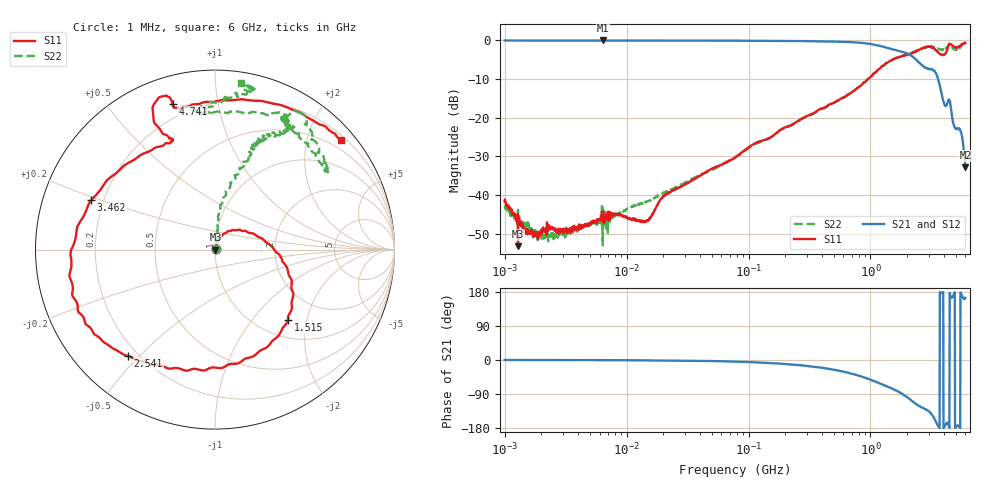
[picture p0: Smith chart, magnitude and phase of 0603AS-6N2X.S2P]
!s-Parameter Generated by FASTRON Sdn. Bhd.
!FASTRON P/N : 0603AS-6N2X
!Keysight Technologies: E5071C_MY46733604_B.14.02
!Date: Tue Nov 21 15:09:04 2023
!Version  :Rev01  Tue Nov 21 15:09:04 2023
!Data & Calibration Information:
!Freq  S11:SOLT2(ON)  S21:SOLT2(ON)  S12:SOLT2(ON)  S22:SOLT2(ON)
!PortZ  Port1:50+j0  Port2:50+j0
!When reading reference impedance value at option line is always used.
! Remarks : This data is being provided solely for informational purposes.
# Hz S dB R 50
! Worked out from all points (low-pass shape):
!   1601 points, 1 MHz to 6 GHz, reference 50 ohm
!   highest |S21| = -0.01 dB at 6.378 MHz (marker M1); lowest = -32.8 dB at 6 GHz (marker M2)
!   |S21| within 3 dB of the highest: start of sweep to 1.829 GHz
!   lowest |S11| = -53.2 dB at 1.288 MHz (marker M3), VSWR 1.00, Z = 50.2 - j0.0158 ohm
!   |S11| at or under -10 dB: start of sweep to 953.5 MHz
!   |S22| runs from -53.0 to -0.5 dB; largest |S21 - S12| = 0.01
!   S11 on the Smith chart (normalised r, x): 1 MHz: 1.02, +0.01; 1.515 GHz: 1.35, -1.55; 2.541 GHz: 0.16, -0.46; 3.462 GHz: 0.15, +0.19; 4.741 GHz: 0.13, +0.74; 6 GHz: 0.30, +2.64
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1000000  -41.61 20.7  -0.03 0.1  -0.05 0.2  -42.82 27.1
1287650  -53.18 -4.1  -0.05 -0.0  -0.04 0.1  -43.78 5.1
2105185  -49.18 39.2  -0.04 -0.1  -0.05 -0.0  -50.93 47.0
4277066  -48.43 44.9  -0.04 -0.2  -0.04 -0.2  -48.53 52.3
6378092  -46.48 62.7  -0.01 -0.4  -0.07 -0.5  -52.95 65.8
1.425742e7  -46.94 69.8  -0.04 -0.8  -0.05 -0.9  -41.84 49.7
1.823719e7  -42.03 65.3  -0.04 -1.1  -0.05 -1.0  -40.07 62.1
7.757876e7  -30.27 70.8  -0.07 -4.2  -0.08 -4.2  -30.27 73.7
3.307917e8  -18.99 56.3  -0.20 -17.0  -0.21 -17.0  -19.17 82.6
8.417592e8  -11.54 14.3  -0.64 -43.5  -0.64 -43.5  -11.51 81.2
1.414819e9  -5.49 -36.2  -2.04 -71.9  -2.05 -72.0  -5.51 69.7
1.515084e9  -4.97 -43.9  -2.31 -76.2  -2.32 -76.2  -4.98 69.2
2.045604e9  -3.63 -89.2  -3.55 -100.4  -3.57 -100.4  -3.49 68.9
2.540942e9  -2.32 -129.3  -5.89 -122.2  -5.89 -122.1  -2.32 60.8
3.00975e9  -1.55 -156.1  -7.40 -135.2  -7.36 -135.2  -1.57 62.7
3.462469e9  -2.58 158.3  -8.73 -164.9  -8.71 -165.2  -1.92 53.7
4.090194e9  -3.51 112.1  -16.85 -173.0  -16.88 -173.3  -2.27 38.8
4.405148e9  -1.00 111.4  -15.28 -175.9  -15.31 -176.2  -1.21 53.9
4.740907e9  -1.45 106.2  -21.06 169.0  -21.11 168.8  -1.99 74.7
5.188584e9  -1.77 96.4  -22.84 -173.5  -22.87 -173.5  -2.39 95.5
5.552322e9  -1.15 68.0  -23.86 174.0  -23.88 174.0  -1.43 84.8
6e9  -0.65 41.1  -32.82 164.1  -32.82 164.0  -0.53 81.2
